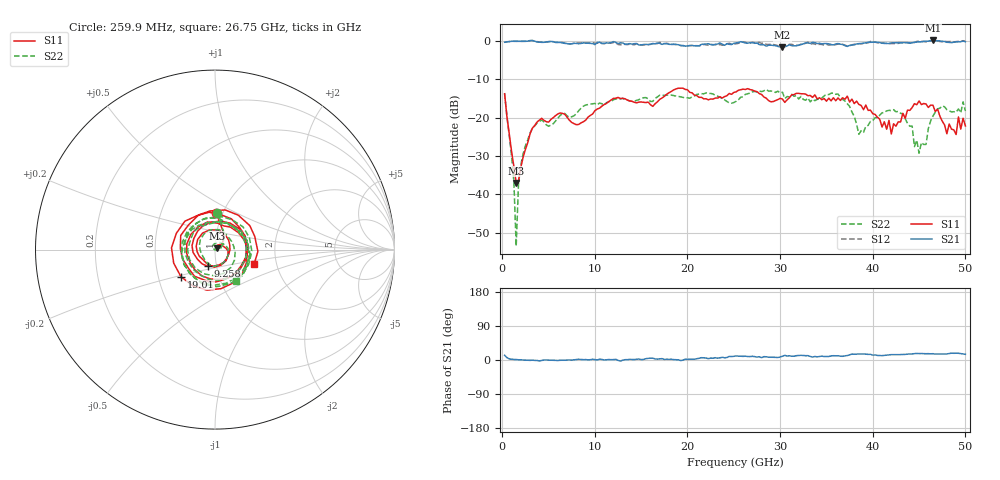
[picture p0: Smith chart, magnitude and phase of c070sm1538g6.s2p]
! 12/1/2022 12:16:31 PM
! D:\C070SM1538G6.S2P
! CHANNEL.1
! TR.MEASUREMENT
! CORRECTED.DATA
# GHZ S RI R 50.0
! FREQ.GHZ  S11RE  S11IM  S21RE  S21IM  S12RE  S12IM  S22RE  S22IM
!; PortSelection: Port_12
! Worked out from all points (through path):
!   200 points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, 259.9 MHz to 50 GHz, reference 50 ohm
!   highest |S21| = 0.14 dB at 46.5 GHz (marker M1); lowest = -1.7 dB at 30.25 GHz (marker M2)
!   lowest |S11| = -37.0 dB at 1.51 GHz (marker M3), VSWR 1.03, Z = 51.2 + j0.811 ohm
!   |S11| at or under -10 dB: start of sweep to end of sweep
!   |S22| runs from -53.5 to -12.6 dB; largest |S21 - S12| = 0.066
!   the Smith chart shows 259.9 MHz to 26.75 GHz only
!   S11 on the Smith chart (normalised r, x): 259.9 MHz: 0.93, +0.40; 9.258 GHz: 0.91, -0.17; 19.01 GHz: 0.65, -0.21; 26.75 GHz: 1.53, -0.27
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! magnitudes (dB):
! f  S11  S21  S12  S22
! 259.9 MHz  -13.8  -0.3  -0.3  -13.7
! 1.26 GHz  -32.7  -0.1  -0.1  -36.6
! 1.51 GHz  -37.0  -0.1  -0.1  -53.5
! 1.76 GHz  -36.5  -0.1  -0.1  -37.2
! 3.009 GHz  -24.2  0.1  0.1  -24.0
! 8.758 GHz  -21.1  -0.5  -0.5  -17.0
! 9.258 GHz  -19.9  -0.6  -0.6  -16.6
! 17.01 GHz  -15.2  -0.6  -0.3  -14.1
! 19.01 GHz  -12.3  -1.0  -0.9  -14.5
! 25.25 GHz  -13.3  -0.5  -0.7  -15.7
! 26.75 GHz  -12.7  -0.5  -0.6  -13.6
! 30.25 GHz  -15.2  -1.7  -1.6  -13.4
! 33.5 GHz  -14.7  -0.4  -0.7  -15.2
! 36.25 GHz  -14.8  -0.7  -0.8  -13.8
! 38.5 GHz  -16.5  -0.7  -0.7  -24.3
! 41.75 GHz  -20.7  -0.6  -0.8  -18.1
! 42 GHz  -24.2  -0.5  -0.7  -18.2
! 44.25 GHz  -17.3  -0.5  -0.6  -22.2
! 45 GHz  -15.6  -0.3  0.0  -29.3
! 46.5 GHz  -16.8  0.1  0.1  -19.6
! 48 GHz  -24.2  -0.3  -0.2  -17.9
! 50 GHz  -22.1  -0.2  -0.1  -18.3
